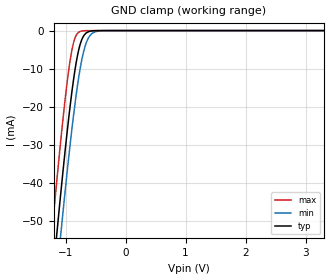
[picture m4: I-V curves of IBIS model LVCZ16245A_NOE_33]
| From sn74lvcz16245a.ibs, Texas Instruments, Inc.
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[Model]   LVCZ16245A_NOE_33
Model_type  Input
Vinl = 0.8
Vinh = 2
| variable   typ   min   max
C_comp   1.44pF   1.02pF   1.90pF
[Temperature Range]   40   100   -40
| Ambient temperature   25   85   -40
[Voltage range]   3.3   3   3.6
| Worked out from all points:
|   GND clamp passes 1 mA (typ) near -0.68 V on its own axis
[GND Clamp]
| LVCZ16245A_NOE_33
|   Voltage   I(typ)   I(min)   I(max)
-5V       -776.3mA   -784.3mA   -766.7mA
-1.25V    -71.03mA   -81.88mA   -57.11mA
-1.22V    -65.92mA   -76.78mA   -51.96mA
-1.145V   -53.37mA   -64.25mA   -39.37mA
-1.08V    -42.85mA   -53.67mA   -28.94mA
-980mV    -27.63mA   -38.14mA   -14.46mA
-900mV    -16.83mA   -26.68mA   -5.63mA
-835mV    -9.584mA   -18.33mA   -1.666mA
-755mV    -3.546mA   -9.857mA   -229.4uA
-630mV    -388.6uA   -2.274mA   -7.794uA
-435mV    -7.673uA   -98.77uA   -37.99nA
3.3V      1.114nA    59.61nA    6.193pA
